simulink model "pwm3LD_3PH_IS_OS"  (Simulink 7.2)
settings: Solver=ode3  SolverMode=SingleTasking  StartTime=0.0  StopTime=0.1  FixedStep=10e-6  MaxStep=1e-4  RelTol=1e-3
PostLoadFcn:
  | INIT_PWM_3L
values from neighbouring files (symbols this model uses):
  VDC = 600    [INIT_PWM_2L.m]    (also in INIT_PWM_3L.m = 1200; INIT_PWM_Con.m = 1200; INIT_B6_2L_3Ph_IGBT_OS.m; INIT_B6_3L_3Ph_IGBT_OS.m = 1000)

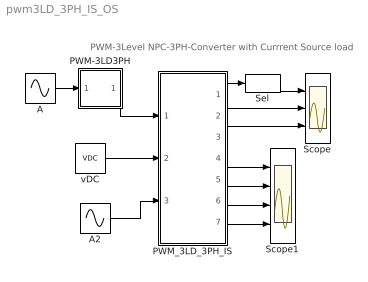
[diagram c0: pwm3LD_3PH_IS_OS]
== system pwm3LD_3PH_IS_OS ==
  note: PWM-3Level NPC-3PH-Converter with Currrent Source load
  A : Sin  Amplitude=.8  Frequency=2*pi*50  Phase="[0  -2*pi/3  -4*pi/3 ]"  SampleTime=0
  A2 : Sin  Amplitude=500  Frequency=2*pi*50  Phase="[0  -2*pi/3 ]"  SampleTime=0
  PWM-3LD3PH : Subsystem  mask(PWM-3LD3PH){FT=900, PHT=0, A=0.5, O1=0.5, O2=-0.5, DT=1e-6}
      mask prompts: FT "Frequency of Trian Sig."; PHT "Phase Angle of Trian. Sig."; A "Amplitude of Trian. Sig."; O1 "Offset of 1st Trian"; O2 "Offset of 2nd Trian."; DT "Dead Time"
      mask help: Pulse Width Modulation for 3 Phase 3 Level Neutral point clamped Converter
  PWM_3LD_3PH_IS : Subsystem
  Scope : Scope  NumInputPorts=3
  Scope1 : Scope  NumInputPorts=4
  Sel : Selector  InputPortWidth=3  IndexOptions=Index vector (dialog)  Indices=[1 ]  OutputSizes=1
  vDC : Constant  Value=VDC  OutDataType=sfix(16)  OutScaling=2^0
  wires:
  A/1 -> PWM-3LD3PH/1(In1)
  A2/1 -> PWM_3LD_3PH_IS/3(I_AB)
  vDC/1 -> PWM_3LD_3PH_IS/2(vDC)
  PWM-3LD3PH/1(Out1) -> PWM_3LD_3PH_IS/1(Sw)
  PWM_3LD_3PH_IS/4("iT1, iD1,vT1") -> Scope1/1
  PWM_3LD_3PH_IS/5("iT2, iD2,vT2") -> Scope1/2
  PWM_3LD_3PH_IS/6(iD5,vD5) -> Scope1/3
  PWM_3LD_3PH_IS/1(vABC) -> Sel/1
  PWM_3LD_3PH_IS/2(iABC) -> Scope/2
  PWM_3LD_3PH_IS/3(vAB) -> Scope/3
  PWM_3LD_3PH_IS/7(iDC1,iDC2) -> Scope1/4
  Sel/1 -> Scope/1

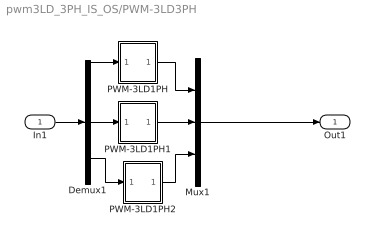
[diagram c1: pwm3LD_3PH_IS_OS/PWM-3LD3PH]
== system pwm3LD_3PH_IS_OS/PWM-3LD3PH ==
  In1 : Inport  OutDataType=sfix(16)  OutScaling=2^0
  Demux1 : Demux  Outputs=3
  Mux1 : Mux  Inputs=3
  PWM-3LD1PH : Subsystem  mask(PWM-3LD_1PH){FT=FT, PHT=PHT, A=A, O1=O1, O2=O2, DT=DT}
      mask prompts: FT "Frequency of Trian Sig."; PHT "Phase Angle of Trian. Sig."; A "Amplitude of Trian. Sig."; O1 "Offset of 1st Trian"; O2 "Offset of 2nd Trian."; DT "Dead Time"
      mask help: Pulse Width Modulation for 1 Leg of 3 Level Neutral point clamped Converter
  PWM-3LD1PH1 : Subsystem  mask(PWM-3LD_1PH){FT=FT, PHT=PHT, A=A, O1=O1, O2=O2, DT=DT}
      mask prompts: FT "Frequency of Trian Sig."; PHT "Phase Angle of Trian. Sig."; A "Amplitude of Trian. Sig."; O1 "Offset of 1st Trian"; O2 "Offset of 2nd Trian."; DT "Dead Time"
      mask help: Pulse Width Modulation for 1 Leg of 3 Level Neutral point clamped Converter
  PWM-3LD1PH2 : Subsystem  mask(PWM-3LD_1PH){FT=FT, PHT=PHT, A=A, O1=O1, O2=O2, DT=DT}
      mask prompts: FT "Frequency of Trian Sig."; PHT "Phase Angle of Trian. Sig."; A "Amplitude of Trian. Sig."; O1 "Offset of 1st Trian"; O2 "Offset of 2nd Trian."; DT "Dead Time"
      mask help: Pulse Width Modulation for 1 Leg of 3 Level Neutral point clamped Converter
  Out1 : Outport
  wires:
  In1/1 -> Demux1/1
  Demux1/3 -> PWM-3LD1PH2/1(In1)
  Demux1/2 -> PWM-3LD1PH1/1(In1)
  Demux1/1 -> PWM-3LD1PH/1(In1)
  Mux1/1 -> Out1/1
  PWM-3LD1PH2/1(Out1) -> Mux1/3
  PWM-3LD1PH1/1(Out1) -> Mux1/2
  PWM-3LD1PH/1(Out1) -> Mux1/1

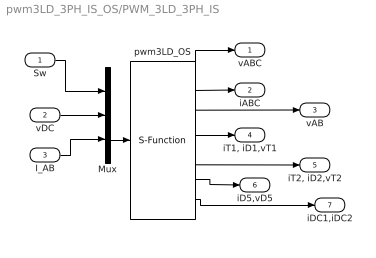
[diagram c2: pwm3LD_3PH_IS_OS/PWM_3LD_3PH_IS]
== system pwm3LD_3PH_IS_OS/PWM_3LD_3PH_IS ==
  Sw : Inport  OutDataType=sfix(16)  OutScaling=2^0
  vDC : Inport  Port=2  OutDataType=sfix(16)  OutScaling=2^0
  I_AB : Inport  Port=3  OutDataType=sfix(16)  OutScaling=2^0
  Mux : Mux  Inputs="[12  1  2]"
  pwm3LD_OS : S-Function  FunctionName=s_pwm_3LD_3PH_IS_OS  Parameters=0  EnableBusSupport=off
  vABC : Outport  OutDataType=sfix(16)  OutScaling=2^0
  iABC : Outport  Port=2  OutDataType=sfix(16)  OutScaling=2^0
  vAB : Outport  Port=3  OutDataType=sfix(16)  OutScaling=2^0
  "iT1, iD1,vT1" : Outport  Port=4  OutDataType=sfix(16)  OutScaling=2^0
  "iT2, iD2,vT2" : Outport  Port=5  OutDataType=sfix(16)  OutScaling=2^0
  iD5,vD5 : Outport  Port=6  OutDataType=sfix(16)  OutScaling=2^0
  iDC1,iDC2 : Outport  Port=7  OutDataType=sfix(16)  OutScaling=2^0
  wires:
  Sw/1 -> Mux/1
  vDC/1 -> Mux/2
  Mux/1 -> pwm3LD_OS/1
  I_AB/1 -> Mux/3
  pwm3LD_OS/1 -> vABC/1
  pwm3LD_OS/4 -> "iT1, iD1,vT1"/1
  pwm3LD_OS/2 -> iABC/1
  pwm3LD_OS/3 -> vAB/1
  pwm3LD_OS/5 -> "iT2, iD2,vT2"/1
  pwm3LD_OS/6 -> iD5,vD5/1
  pwm3LD_OS/7 -> iDC1,iDC2/1

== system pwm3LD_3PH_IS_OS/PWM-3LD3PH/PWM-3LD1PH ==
  In1 : Inport  OutDataType=sfix(16)  OutScaling=2^0
  Mux : Mux
  SS : Subsystem
  SS1 : Subsystem
  Out1 : Outport
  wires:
  In1/1 -> SS1/1(I1), SS/1(I1)
  SS1/1(O1) -> Mux/2
  SS/2(O2) -> Mux/3
  Mux/1 -> Out1/1
  SS/1(O1) -> Mux/1
  SS1/2(O2) -> Mux/4

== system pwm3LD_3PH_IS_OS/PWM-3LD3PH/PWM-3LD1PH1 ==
  In1 : Inport  OutDataType=sfix(16)  OutScaling=2^0
  Mux : Mux
  SS : Subsystem
  SS1 : Subsystem
  Out1 : Outport
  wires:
  SS1/2(O2) -> Mux/4
  SS/1(O1) -> Mux/1
  Mux/1 -> Out1/1
  SS/2(O2) -> Mux/3
  SS1/1(O1) -> Mux/2
  In1/1 -> SS/1(I1), SS1/1(I1)

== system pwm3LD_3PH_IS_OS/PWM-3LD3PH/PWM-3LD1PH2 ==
  In1 : Inport  OutDataType=sfix(16)  OutScaling=2^0
  Mux : Mux
  SS : Subsystem
  SS1 : Subsystem
  Out1 : Outport
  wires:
  In1/1 -> SS1/1(I1), SS/1(I1)
  SS1/1(O1) -> Mux/2
  SS/2(O2) -> Mux/3
  Mux/1 -> Out1/1
  SS/1(O1) -> Mux/1
  SS1/2(O2) -> Mux/4

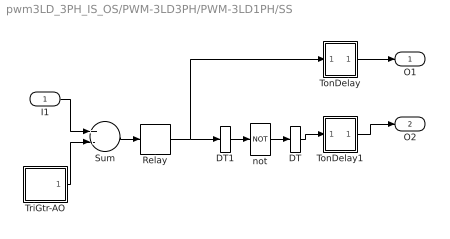
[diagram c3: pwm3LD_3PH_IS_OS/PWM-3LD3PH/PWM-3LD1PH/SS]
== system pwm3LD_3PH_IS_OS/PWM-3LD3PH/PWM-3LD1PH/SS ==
  I1 : Inport  OutDataType=sfix(16)  OutScaling=2^0
  DT : DataTypeConversion
  DT1 : DataTypeConversion
  Relay : Relay  OutDataType=sfix(16)  OutScaling=2^0
  Sum : Sum  Inputs=+-  OutDataType=sfix(16)  OutScaling=2^0
  TonDelay : Subsystem  mask(TonDelay){DT=DT}
      mask prompts: DT "Dead Time"
      mask help: Turn on dead time to protect against short circuit of the converter leg
  TonDelay1 : Subsystem  mask(TonDelay){DT=DT}
      mask prompts: DT "Dead Time"
      mask help: Turn on dead time to protect against short circuit of the converter leg
  TriGtr-AO : Subsystem  mask(TriGtr-AO){A=A, O=O1, T=1/FT, Td=PHT/FT/180}
      mask prompts: A "Amplitude"; O "Offset"; T "Period Time"; Td "Time Delay"
      mask help: Triangular Wave Generator with variable time delay, variable amplitude and offset
  not : Logic  Operator=NOT  Inputs=1
  O1 : Outport  InitialOutput=0
  O2 : Outport  Port=2  InitialOutput=0
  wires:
  TonDelay/1(s1d) -> O1/1
  Relay/1 -> TonDelay/1(s1), DT1/1
  TonDelay1/1(s1d) -> O2/1
  not/1 -> DT/1
  Sum/1 -> Relay/1
  TriGtr-AO/1(Out1) -> Sum/2
  I1/1 -> Sum/1
  DT/1 -> TonDelay1/1(s1)
  DT1/1 -> not/1

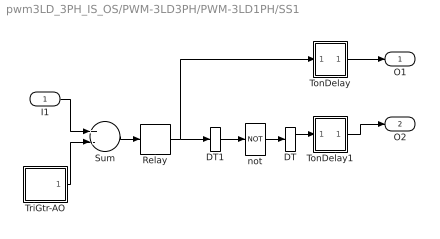
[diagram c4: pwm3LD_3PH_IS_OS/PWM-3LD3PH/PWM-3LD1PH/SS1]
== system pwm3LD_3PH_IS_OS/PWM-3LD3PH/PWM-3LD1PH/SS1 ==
  I1 : Inport  OutDataType=sfix(16)  OutScaling=2^0
  DT : DataTypeConversion
  DT1 : DataTypeConversion
  Relay : Relay  OutDataType=sfix(16)  OutScaling=2^0
  Sum : Sum  Inputs=+-  OutDataType=sfix(16)  OutScaling=2^0
  TonDelay : Subsystem  mask(TonDelay){DT=DT}
      mask prompts: DT "Dead Time"
      mask help: Turn on dead time to protect against short circuit of the converter leg
  TonDelay1 : Subsystem  mask(TonDelay){DT=DT}
      mask prompts: DT "Dead Time"
      mask help: Turn on dead time to protect against short circuit of the converter leg
  TriGtr-AO : Subsystem  mask(TriGtr-AO){A=A, O=O2, T=1/FT, Td=PHT/FT/180}
      mask prompts: A "Amplitude"; O "Offset"; T "Period Time"; Td "Time Delay"
      mask help: Triangular Wave Generator with variable time delay, variable amplitude and offset
  not : Logic  Operator=NOT  Inputs=1
  O1 : Outport  InitialOutput=0
  O2 : Outport  Port=2  InitialOutput=0
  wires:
  TonDelay/1(s1d) -> O1/1
  Relay/1 -> TonDelay/1(s1), DT1/1
  TonDelay1/1(s1d) -> O2/1
  not/1 -> DT/1
  Sum/1 -> Relay/1
  TriGtr-AO/1(Out1) -> Sum/2
  I1/1 -> Sum/1
  DT/1 -> TonDelay1/1(s1)
  DT1/1 -> not/1

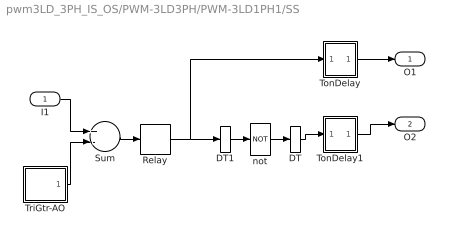
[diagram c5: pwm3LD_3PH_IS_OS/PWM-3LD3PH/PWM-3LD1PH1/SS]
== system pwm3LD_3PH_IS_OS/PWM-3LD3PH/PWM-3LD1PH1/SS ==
  I1 : Inport  OutDataType=sfix(16)  OutScaling=2^0
  DT : DataTypeConversion
  DT1 : DataTypeConversion
  Relay : Relay  OutDataType=sfix(16)  OutScaling=2^0
  Sum : Sum  Inputs=+-  OutDataType=sfix(16)  OutScaling=2^0
  TonDelay : Subsystem  mask(TonDelay){DT=DT}
      mask prompts: DT "Dead Time"
      mask help: Turn on dead time to protect against short circuit of the converter leg
  TonDelay1 : Subsystem  mask(TonDelay){DT=DT}
      mask prompts: DT "Dead Time"
      mask help: Turn on dead time to protect against short circuit of the converter leg
  TriGtr-AO : Subsystem  mask(TriGtr-AO){A=A, O=O1, T=1/FT, Td=PHT/FT/180}
      mask prompts: A "Amplitude"; O "Offset"; T "Period Time"; Td "Time Delay"
      mask help: Triangular Wave Generator with variable time delay, variable amplitude and offset
  not : Logic  Operator=NOT  Inputs=1
  O1 : Outport  InitialOutput=0
  O2 : Outport  Port=2  InitialOutput=0
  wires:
  DT1/1 -> not/1
  DT/1 -> TonDelay1/1(s1)
  I1/1 -> Sum/1
  TriGtr-AO/1(Out1) -> Sum/2
  Sum/1 -> Relay/1
  not/1 -> DT/1
  TonDelay1/1(s1d) -> O2/1
  Relay/1 -> DT1/1, TonDelay/1(s1)
  TonDelay/1(s1d) -> O1/1

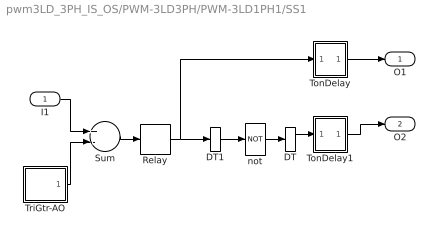
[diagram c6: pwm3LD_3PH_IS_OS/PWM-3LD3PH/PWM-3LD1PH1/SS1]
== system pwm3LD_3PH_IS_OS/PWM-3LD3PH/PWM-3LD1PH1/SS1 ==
  I1 : Inport  OutDataType=sfix(16)  OutScaling=2^0
  DT : DataTypeConversion
  DT1 : DataTypeConversion
  Relay : Relay  OutDataType=sfix(16)  OutScaling=2^0
  Sum : Sum  Inputs=+-  OutDataType=sfix(16)  OutScaling=2^0
  TonDelay : Subsystem  mask(TonDelay){DT=DT}
      mask prompts: DT "Dead Time"
      mask help: Turn on dead time to protect against short circuit of the converter leg
  TonDelay1 : Subsystem  mask(TonDelay){DT=DT}
      mask prompts: DT "Dead Time"
      mask help: Turn on dead time to protect against short circuit of the converter leg
  TriGtr-AO : Subsystem  mask(TriGtr-AO){A=A, O=O2, T=1/FT, Td=PHT/FT/180}
      mask prompts: A "Amplitude"; O "Offset"; T "Period Time"; Td "Time Delay"
      mask help: Triangular Wave Generator with variable time delay, variable amplitude and offset
  not : Logic  Operator=NOT  Inputs=1
  O1 : Outport  InitialOutput=0
  O2 : Outport  Port=2  InitialOutput=0
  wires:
  DT1/1 -> not/1
  DT/1 -> TonDelay1/1(s1)
  I1/1 -> Sum/1
  TriGtr-AO/1(Out1) -> Sum/2
  Sum/1 -> Relay/1
  not/1 -> DT/1
  TonDelay1/1(s1d) -> O2/1
  Relay/1 -> DT1/1, TonDelay/1(s1)
  TonDelay/1(s1d) -> O1/1

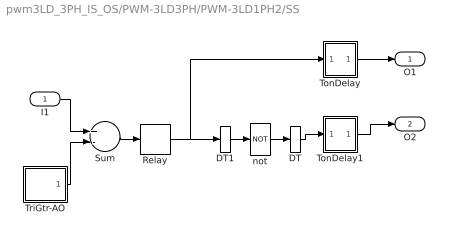
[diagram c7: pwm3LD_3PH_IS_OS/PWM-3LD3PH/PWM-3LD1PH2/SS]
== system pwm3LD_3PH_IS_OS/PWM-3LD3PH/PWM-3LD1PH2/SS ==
  I1 : Inport  OutDataType=sfix(16)  OutScaling=2^0
  DT : DataTypeConversion
  DT1 : DataTypeConversion
  Relay : Relay  OutDataType=sfix(16)  OutScaling=2^0
  Sum : Sum  Inputs=+-  OutDataType=sfix(16)  OutScaling=2^0
  TonDelay : Subsystem  mask(TonDelay){DT=DT}
      mask prompts: DT "Dead Time"
      mask help: Turn on dead time to protect against short circuit of the converter leg
  TonDelay1 : Subsystem  mask(TonDelay){DT=DT}
      mask prompts: DT "Dead Time"
      mask help: Turn on dead time to protect against short circuit of the converter leg
  TriGtr-AO : Subsystem  mask(TriGtr-AO){A=A, O=O1, T=1/FT, Td=PHT/FT/180}
      mask prompts: A "Amplitude"; O "Offset"; T "Period Time"; Td "Time Delay"
      mask help: Triangular Wave Generator with variable time delay, variable amplitude and offset
  not : Logic  Operator=NOT  Inputs=1
  O1 : Outport  InitialOutput=0
  O2 : Outport  Port=2  InitialOutput=0
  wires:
  TonDelay/1(s1d) -> O1/1
  Relay/1 -> TonDelay/1(s1), DT1/1
  TonDelay1/1(s1d) -> O2/1
  not/1 -> DT/1
  Sum/1 -> Relay/1
  TriGtr-AO/1(Out1) -> Sum/2
  I1/1 -> Sum/1
  DT/1 -> TonDelay1/1(s1)
  DT1/1 -> not/1

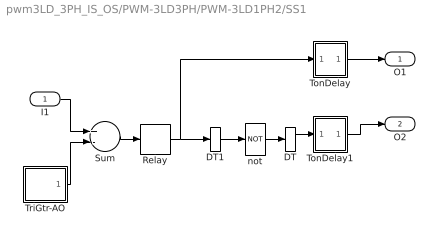
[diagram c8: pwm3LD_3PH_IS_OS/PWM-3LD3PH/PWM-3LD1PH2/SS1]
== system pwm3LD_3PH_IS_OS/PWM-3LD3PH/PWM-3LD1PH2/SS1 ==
  I1 : Inport  OutDataType=sfix(16)  OutScaling=2^0
  DT : DataTypeConversion
  DT1 : DataTypeConversion
  Relay : Relay  OutDataType=sfix(16)  OutScaling=2^0
  Sum : Sum  Inputs=+-  OutDataType=sfix(16)  OutScaling=2^0
  TonDelay : Subsystem  mask(TonDelay){DT=DT}
      mask prompts: DT "Dead Time"
      mask help: Turn on dead time to protect against short circuit of the converter leg
  TonDelay1 : Subsystem  mask(TonDelay){DT=DT}
      mask prompts: DT "Dead Time"
      mask help: Turn on dead time to protect against short circuit of the converter leg
  TriGtr-AO : Subsystem  mask(TriGtr-AO){A=A, O=O2, T=1/FT, Td=PHT/FT/180}
      mask prompts: A "Amplitude"; O "Offset"; T "Period Time"; Td "Time Delay"
      mask help: Triangular Wave Generator with variable time delay, variable amplitude and offset
  not : Logic  Operator=NOT  Inputs=1
  O1 : Outport  InitialOutput=0
  O2 : Outport  Port=2  InitialOutput=0
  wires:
  TonDelay/1(s1d) -> O1/1
  Relay/1 -> TonDelay/1(s1), DT1/1
  TonDelay1/1(s1d) -> O2/1
  not/1 -> DT/1
  Sum/1 -> Relay/1
  TriGtr-AO/1(Out1) -> Sum/2
  I1/1 -> Sum/1
  DT/1 -> TonDelay1/1(s1)
  DT1/1 -> not/1

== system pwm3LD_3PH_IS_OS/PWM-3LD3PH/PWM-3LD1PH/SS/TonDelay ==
  s1 : Inport  Orientation=down  OutDataType=sfix(16)  OutScaling=2^0
  Int : Integrator  ExternalReset=falling
  Rel1 : Relay  OnSwitchValue=DT  OutDataType=sfix(16)  OutScaling=2^0
  s1d : Outport  InitialOutput=0
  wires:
  Rel1/1 -> s1d/1
  s1/1 -> Int/1, Int/2
  Int/1 -> Rel1/1

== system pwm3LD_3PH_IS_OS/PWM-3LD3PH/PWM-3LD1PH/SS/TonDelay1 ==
  s1 : Inport  Orientation=down  OutDataType=sfix(16)  OutScaling=2^0
  Int : Integrator  ExternalReset=falling
  Rel1 : Relay  OnSwitchValue=DT  OutDataType=sfix(16)  OutScaling=2^0
  s1d : Outport  InitialOutput=0
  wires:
  Rel1/1 -> s1d/1
  s1/1 -> Int/1, Int/2
  Int/1 -> Rel1/1

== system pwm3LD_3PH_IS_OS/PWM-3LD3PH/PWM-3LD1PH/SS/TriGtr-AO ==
  Ampl. : Gain  Gain=A  ParameterDataType=sfix(16)  ParameterScaling=2^0  OutDataType=sfix(16)  OutScaling=2^0
  Offset : Constant  Value=O  OutDataType=sfix(16)  OutScaling=2^0
  Sum : Sum  OutDataType=sfix(16)  OutScaling=2^0
  TriGtr1 : Subsystem  mask(TriGtr){T=T, Td=Td}
      mask prompts: T "Period Time"; Td "Time Delay"
      mask help: Triangular Wave Generator with variable time delay
  Out1 : Outport
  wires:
  Sum/1 -> Out1/1
  Ampl./1 -> Sum/1
  TriGtr1/1(O) -> Ampl./1
  Offset/1 -> Sum/2

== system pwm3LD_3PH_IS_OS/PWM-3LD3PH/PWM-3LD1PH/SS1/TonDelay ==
  s1 : Inport  Orientation=down  OutDataType=sfix(16)  OutScaling=2^0
  Int : Integrator  ExternalReset=falling
  Rel1 : Relay  OnSwitchValue=DT  OutDataType=sfix(16)  OutScaling=2^0
  s1d : Outport  InitialOutput=0
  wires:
  Rel1/1 -> s1d/1
  s1/1 -> Int/1, Int/2
  Int/1 -> Rel1/1

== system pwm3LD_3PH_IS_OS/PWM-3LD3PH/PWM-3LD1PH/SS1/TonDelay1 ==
  s1 : Inport  Orientation=down  OutDataType=sfix(16)  OutScaling=2^0
  Int : Integrator  ExternalReset=falling
  Rel1 : Relay  OnSwitchValue=DT  OutDataType=sfix(16)  OutScaling=2^0
  s1d : Outport  InitialOutput=0
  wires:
  Rel1/1 -> s1d/1
  s1/1 -> Int/1, Int/2
  Int/1 -> Rel1/1

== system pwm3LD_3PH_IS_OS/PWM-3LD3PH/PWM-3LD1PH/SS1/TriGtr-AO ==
  Ampl. : Gain  Gain=A  ParameterDataType=sfix(16)  ParameterScaling=2^0  OutDataType=sfix(16)  OutScaling=2^0
  Offset : Constant  Value=O  OutDataType=sfix(16)  OutScaling=2^0
  Sum : Sum  OutDataType=sfix(16)  OutScaling=2^0
  TriGtr1 : Subsystem  mask(TriGtr){T=T, Td=Td}
      mask prompts: T "Period Time"; Td "Time Delay"
      mask help: Triangular Wave Generator with variable time delay
  Out1 : Outport
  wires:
  Offset/1 -> Sum/2
  TriGtr1/1(O) -> Ampl./1
  Ampl./1 -> Sum/1
  Sum/1 -> Out1/1

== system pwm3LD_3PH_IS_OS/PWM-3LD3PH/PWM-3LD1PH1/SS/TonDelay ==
  s1 : Inport  Orientation=down  OutDataType=sfix(16)  OutScaling=2^0
  Int : Integrator  ExternalReset=falling
  Rel1 : Relay  OnSwitchValue=DT  OutDataType=sfix(16)  OutScaling=2^0
  s1d : Outport  InitialOutput=0
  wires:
  Int/1 -> Rel1/1
  s1/1 -> Int/2, Int/1
  Rel1/1 -> s1d/1

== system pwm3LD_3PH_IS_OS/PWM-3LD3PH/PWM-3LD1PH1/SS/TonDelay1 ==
  s1 : Inport  Orientation=down  OutDataType=sfix(16)  OutScaling=2^0
  Int : Integrator  ExternalReset=falling
  Rel1 : Relay  OnSwitchValue=DT  OutDataType=sfix(16)  OutScaling=2^0
  s1d : Outport  InitialOutput=0
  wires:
  Int/1 -> Rel1/1
  s1/1 -> Int/2, Int/1
  Rel1/1 -> s1d/1

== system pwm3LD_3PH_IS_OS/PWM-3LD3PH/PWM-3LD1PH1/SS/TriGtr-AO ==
  Ampl. : Gain  Gain=A  ParameterDataType=sfix(16)  ParameterScaling=2^0  OutDataType=sfix(16)  OutScaling=2^0
  Offset : Constant  Value=O  OutDataType=sfix(16)  OutScaling=2^0
  Sum : Sum  OutDataType=sfix(16)  OutScaling=2^0
  TriGtr1 : Subsystem  mask(TriGtr){T=T, Td=Td}
      mask prompts: T "Period Time"; Td "Time Delay"
      mask help: Triangular Wave Generator with variable time delay
  Out1 : Outport
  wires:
  Offset/1 -> Sum/2
  TriGtr1/1(O) -> Ampl./1
  Ampl./1 -> Sum/1
  Sum/1 -> Out1/1

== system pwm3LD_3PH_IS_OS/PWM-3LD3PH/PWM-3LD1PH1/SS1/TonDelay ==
  s1 : Inport  Orientation=down  OutDataType=sfix(16)  OutScaling=2^0
  Int : Integrator  ExternalReset=falling
  Rel1 : Relay  OnSwitchValue=DT  OutDataType=sfix(16)  OutScaling=2^0
  s1d : Outport  InitialOutput=0
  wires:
  Int/1 -> Rel1/1
  s1/1 -> Int/2, Int/1
  Rel1/1 -> s1d/1

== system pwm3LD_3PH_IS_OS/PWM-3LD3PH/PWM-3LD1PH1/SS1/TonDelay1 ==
  s1 : Inport  Orientation=down  OutDataType=sfix(16)  OutScaling=2^0
  Int : Integrator  ExternalReset=falling
  Rel1 : Relay  OnSwitchValue=DT  OutDataType=sfix(16)  OutScaling=2^0
  s1d : Outport  InitialOutput=0
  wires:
  Int/1 -> Rel1/1
  s1/1 -> Int/2, Int/1
  Rel1/1 -> s1d/1

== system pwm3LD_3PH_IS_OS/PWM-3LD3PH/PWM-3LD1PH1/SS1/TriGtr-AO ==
  Ampl. : Gain  Gain=A  ParameterDataType=sfix(16)  ParameterScaling=2^0  OutDataType=sfix(16)  OutScaling=2^0
  Offset : Constant  Value=O  OutDataType=sfix(16)  OutScaling=2^0
  Sum : Sum  OutDataType=sfix(16)  OutScaling=2^0
  TriGtr1 : Subsystem  mask(TriGtr){T=T, Td=Td}
      mask prompts: T "Period Time"; Td "Time Delay"
      mask help: Triangular Wave Generator with variable time delay
  Out1 : Outport
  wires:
  Sum/1 -> Out1/1
  Ampl./1 -> Sum/1
  TriGtr1/1(O) -> Ampl./1
  Offset/1 -> Sum/2

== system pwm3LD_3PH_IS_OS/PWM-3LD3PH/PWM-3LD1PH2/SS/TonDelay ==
  s1 : Inport  Orientation=down  OutDataType=sfix(16)  OutScaling=2^0
  Int : Integrator  ExternalReset=falling
  Rel1 : Relay  OnSwitchValue=DT  OutDataType=sfix(16)  OutScaling=2^0
  s1d : Outport  InitialOutput=0
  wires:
  Rel1/1 -> s1d/1
  s1/1 -> Int/1, Int/2
  Int/1 -> Rel1/1

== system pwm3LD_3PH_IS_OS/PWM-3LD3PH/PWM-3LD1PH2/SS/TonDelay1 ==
  s1 : Inport  Orientation=down  OutDataType=sfix(16)  OutScaling=2^0
  Int : Integrator  ExternalReset=falling
  Rel1 : Relay  OnSwitchValue=DT  OutDataType=sfix(16)  OutScaling=2^0
  s1d : Outport  InitialOutput=0
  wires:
  Rel1/1 -> s1d/1
  s1/1 -> Int/1, Int/2
  Int/1 -> Rel1/1

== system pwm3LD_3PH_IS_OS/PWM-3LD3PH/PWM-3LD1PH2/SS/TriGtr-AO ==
  Ampl. : Gain  Gain=A  ParameterDataType=sfix(16)  ParameterScaling=2^0  OutDataType=sfix(16)  OutScaling=2^0
  Offset : Constant  Value=O  OutDataType=sfix(16)  OutScaling=2^0
  Sum : Sum  OutDataType=sfix(16)  OutScaling=2^0
  TriGtr1 : Subsystem  mask(TriGtr){T=T, Td=Td}
      mask prompts: T "Period Time"; Td "Time Delay"
      mask help: Triangular Wave Generator with variable time delay
  Out1 : Outport
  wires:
  Sum/1 -> Out1/1
  Ampl./1 -> Sum/1
  TriGtr1/1(O) -> Ampl./1
  Offset/1 -> Sum/2

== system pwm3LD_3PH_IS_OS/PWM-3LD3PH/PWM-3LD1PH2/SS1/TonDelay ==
  s1 : Inport  Orientation=down  OutDataType=sfix(16)  OutScaling=2^0
  Int : Integrator  ExternalReset=falling
  Rel1 : Relay  OnSwitchValue=DT  OutDataType=sfix(16)  OutScaling=2^0
  s1d : Outport  InitialOutput=0
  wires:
  Rel1/1 -> s1d/1
  s1/1 -> Int/1, Int/2
  Int/1 -> Rel1/1

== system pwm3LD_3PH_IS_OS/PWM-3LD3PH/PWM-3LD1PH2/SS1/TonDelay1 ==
  s1 : Inport  Orientation=down  OutDataType=sfix(16)  OutScaling=2^0
  Int : Integrator  ExternalReset=falling
  Rel1 : Relay  OnSwitchValue=DT  OutDataType=sfix(16)  OutScaling=2^0
  s1d : Outport  InitialOutput=0
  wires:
  Rel1/1 -> s1d/1
  s1/1 -> Int/1, Int/2
  Int/1 -> Rel1/1

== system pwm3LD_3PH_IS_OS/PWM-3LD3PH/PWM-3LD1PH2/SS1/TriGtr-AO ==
  Ampl. : Gain  Gain=A  ParameterDataType=sfix(16)  ParameterScaling=2^0  OutDataType=sfix(16)  OutScaling=2^0
  Offset : Constant  Value=O  OutDataType=sfix(16)  OutScaling=2^0
  Sum : Sum  OutDataType=sfix(16)  OutScaling=2^0
  TriGtr1 : Subsystem  mask(TriGtr){T=T, Td=Td}
      mask prompts: T "Period Time"; Td "Time Delay"
      mask help: Triangular Wave Generator with variable time delay
  Out1 : Outport
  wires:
  Offset/1 -> Sum/2
  TriGtr1/1(O) -> Ampl./1
  Ampl./1 -> Sum/1
  Sum/1 -> Out1/1

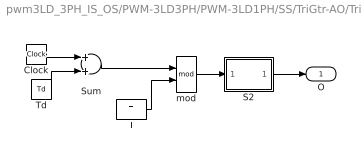
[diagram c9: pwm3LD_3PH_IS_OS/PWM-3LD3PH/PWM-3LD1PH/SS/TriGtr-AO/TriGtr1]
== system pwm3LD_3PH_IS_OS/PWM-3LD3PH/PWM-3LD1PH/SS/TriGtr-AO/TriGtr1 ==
  Clock : Clock
  S2 : Subsystem
  Sum : Sum  OutDataType=sfix(16)  OutScaling=2^0
  T : Constant  Value=T  OutDataType=sfix(16)  OutScaling=2^0
  Td : Constant  Value=Td  OutDataType=sfix(16)  OutScaling=2^0
  mod : Math  Operator=mod
  O : Outport  InitialOutput=0
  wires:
  Td/1 -> Sum/2
  Sum/1 -> mod/1
  T/1 -> mod/2
  Clock/1 -> Sum/1
  S2/1(O1) -> O/1
  mod/1 -> S2/1(I1)

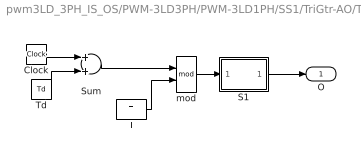
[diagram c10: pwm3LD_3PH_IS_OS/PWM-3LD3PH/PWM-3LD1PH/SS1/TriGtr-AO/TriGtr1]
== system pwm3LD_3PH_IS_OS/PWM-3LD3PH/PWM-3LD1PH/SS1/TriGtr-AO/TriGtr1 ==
  Clock : Clock
  S1 : Subsystem
  Sum : Sum
  T : Constant  Value=T
  Td : Constant  Value=Td
  mod : Math  Operator=mod
  O : Outport  InitialOutput=0
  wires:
  Td/1 -> Sum/2
  Sum/1 -> mod/1
  T/1 -> mod/2
  Clock/1 -> Sum/1
  S1/1(O1) -> O/1
  mod/1 -> S1/1(I1)

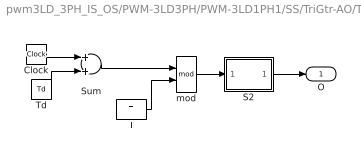
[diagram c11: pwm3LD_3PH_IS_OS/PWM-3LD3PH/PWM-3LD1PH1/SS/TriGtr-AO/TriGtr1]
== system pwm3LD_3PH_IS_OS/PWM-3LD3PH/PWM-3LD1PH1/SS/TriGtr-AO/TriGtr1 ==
  Clock : Clock
  S2 : Subsystem
  Sum : Sum  OutDataType=sfix(16)  OutScaling=2^0
  T : Constant  Value=T  OutDataType=sfix(16)  OutScaling=2^0
  Td : Constant  Value=Td  OutDataType=sfix(16)  OutScaling=2^0
  mod : Math  Operator=mod
  O : Outport  InitialOutput=0
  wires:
  mod/1 -> S2/1(I1)
  S2/1(O1) -> O/1
  Clock/1 -> Sum/1
  T/1 -> mod/2
  Sum/1 -> mod/1
  Td/1 -> Sum/2

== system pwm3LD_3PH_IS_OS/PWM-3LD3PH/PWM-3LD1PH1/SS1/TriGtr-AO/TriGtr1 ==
  Clock : Clock
  S1 : Subsystem
  Sum : Sum
  T : Constant  Value=T
  Td : Constant  Value=Td
  mod : Math  Operator=mod
  O : Outport  InitialOutput=0
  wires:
  mod/1 -> S1/1(I1)
  S1/1(O1) -> O/1
  Clock/1 -> Sum/1
  T/1 -> mod/2
  Sum/1 -> mod/1
  Td/1 -> Sum/2

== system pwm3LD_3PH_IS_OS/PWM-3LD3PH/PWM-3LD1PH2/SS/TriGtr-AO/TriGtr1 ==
  Clock : Clock
  S2 : Subsystem
  Sum : Sum  OutDataType=sfix(16)  OutScaling=2^0
  T : Constant  Value=T  OutDataType=sfix(16)  OutScaling=2^0
  Td : Constant  Value=Td  OutDataType=sfix(16)  OutScaling=2^0
  mod : Math  Operator=mod
  O : Outport  InitialOutput=0
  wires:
  Td/1 -> Sum/2
  Sum/1 -> mod/1
  T/1 -> mod/2
  Clock/1 -> Sum/1
  S2/1(O1) -> O/1
  mod/1 -> S2/1(I1)

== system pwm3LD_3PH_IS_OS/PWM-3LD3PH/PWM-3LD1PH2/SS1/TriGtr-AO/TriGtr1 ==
  Clock : Clock
  S1 : Subsystem
  Sum : Sum
  T : Constant  Value=T
  Td : Constant  Value=Td
  mod : Math  Operator=mod
  O : Outport  InitialOutput=0
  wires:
  Td/1 -> Sum/2
  Sum/1 -> mod/1
  T/1 -> mod/2
  Clock/1 -> Sum/1
  S1/1(O1) -> O/1
  mod/1 -> S1/1(I1)

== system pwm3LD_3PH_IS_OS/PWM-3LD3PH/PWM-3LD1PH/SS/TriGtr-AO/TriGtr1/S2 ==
  I1 : Inport
  Fcn : Fcn  Expr="(u* (u <=T/4) * 4/T)   +  (  (u > T/4) && ( u <=3*T/4) )* ( 1 - (u-T/4) *4/T )   +  ( (u > 3*T/4)&& (u<=T)) * ( ((u -3*T/4)* 4/T )-1 )"
  O1 : Outport
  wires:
  Fcn/1 -> O1/1
  I1/1 -> Fcn/1

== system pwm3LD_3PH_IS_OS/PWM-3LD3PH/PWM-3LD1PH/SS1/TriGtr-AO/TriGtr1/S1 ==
  I1 : Inport
  Fcn : Fcn  Expr="(u* (u <=T/4) * 4/T)   +  (  (u > T/4) && ( u <=3*T/4) )* ( 1 - (u-T/4) *4/T )   +  ( (u > 3*T/4)&& (u<=T)) * ( ((u -3*T/4)* 4/T )-1 )"
  O1 : Outport
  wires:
  I1/1 -> Fcn/1
  Fcn/1 -> O1/1

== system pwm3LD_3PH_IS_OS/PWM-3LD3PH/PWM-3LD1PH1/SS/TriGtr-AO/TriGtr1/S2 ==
  I1 : Inport
  Fcn : Fcn  Expr="(u* (u <=T/4) * 4/T)   +  (  (u > T/4) && ( u <=3*T/4) )* ( 1 - (u-T/4) *4/T )   +  ( (u > 3*T/4)&& (u<=T)) * ( ((u -3*T/4)* 4/T )-1 )"
  O1 : Outport
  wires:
  I1/1 -> Fcn/1
  Fcn/1 -> O1/1

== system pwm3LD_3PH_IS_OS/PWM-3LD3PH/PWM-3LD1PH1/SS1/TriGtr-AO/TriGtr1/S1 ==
  I1 : Inport
  Fcn : Fcn  Expr="(u* (u <=T/4) * 4/T)   +  (  (u > T/4) && ( u <=3*T/4) )* ( 1 - (u-T/4) *4/T )   +  ( (u > 3*T/4)&& (u<=T)) * ( ((u -3*T/4)* 4/T )-1 )"
  O1 : Outport
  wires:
  Fcn/1 -> O1/1
  I1/1 -> Fcn/1

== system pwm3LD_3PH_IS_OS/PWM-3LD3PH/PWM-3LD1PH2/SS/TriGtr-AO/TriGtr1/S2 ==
  I1 : Inport
  Fcn : Fcn  Expr="(u* (u <=T/4) * 4/T)   +  (  (u > T/4) && ( u <=3*T/4) )* ( 1 - (u-T/4) *4/T )   +  ( (u > 3*T/4)&& (u<=T)) * ( ((u -3*T/4)* 4/T )-1 )"
  O1 : Outport
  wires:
  Fcn/1 -> O1/1
  I1/1 -> Fcn/1

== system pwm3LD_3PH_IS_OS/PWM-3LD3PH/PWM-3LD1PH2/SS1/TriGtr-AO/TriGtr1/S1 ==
  I1 : Inport
  Fcn : Fcn  Expr="(u* (u <=T/4) * 4/T)   +  (  (u > T/4) && ( u <=3*T/4) )* ( 1 - (u-T/4) *4/T )   +  ( (u > 3*T/4)&& (u<=T)) * ( ((u -3*T/4)* 4/T )-1 )"
  O1 : Outport
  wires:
  I1/1 -> Fcn/1
  Fcn/1 -> O1/1
